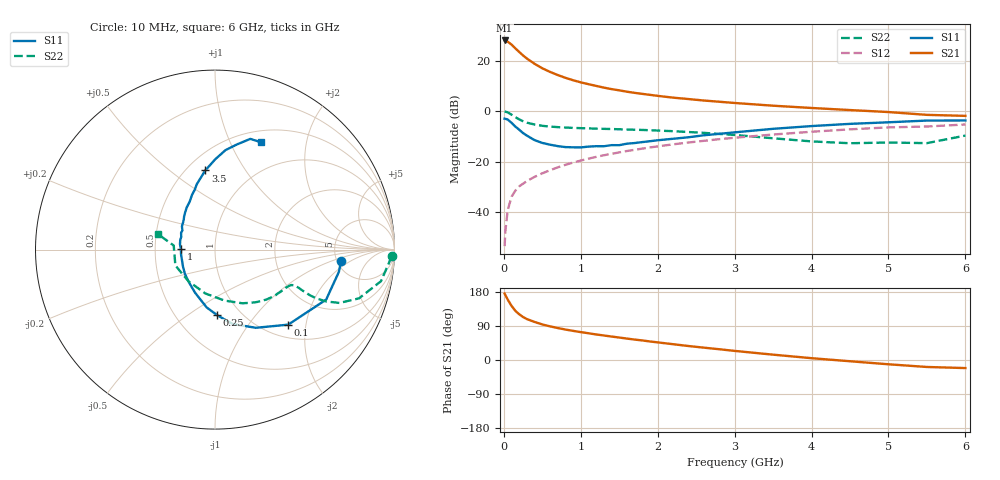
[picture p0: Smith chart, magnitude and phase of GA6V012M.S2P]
! Infineon Technologies  Discrete & RF Semiconductors
! BF775
! Si NPN RF Bipolar Junction Transistor in SOT23
! VCE = 6 V  IC = 12 mA
! Common Emitter S-Parameters:  May  1996
# GHz  S  MA  R  50
!  f  S11  S21  S12  S22
! GHz  MAG  ANG  MAG  ANG  MAG  ANG  MAG  ANG
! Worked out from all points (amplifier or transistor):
!   36 points, 10 MHz to 6 GHz, reference 50 ohm
!   highest |S21| = 28.0 dB at 10 MHz (marker M1)
!   |S21| within 3 dB of that: start of sweep to 145.3 MHz
!   unconditionally stable (mu >= 1): 552.3 MHz to 2.917 GHz
!   at 250 MHz: K = 0.72, MSG = 25.4 dB, |S12| = -28.8 dB
!   at 1.4 GHz: K = 1.10, MAG = 10.9 dB, |S12| = -17.0 dB
!   at 6 GHz: K = 0.91, MSG = 1.7 dB, |S12| = -5.3 dB
!   S11 on the Smith chart (normalised r, x): 10 MHz: 5.42, -1.38; 100 MHz: 1.25, -1.59; 250 MHz: 0.78, -0.66; 1 GHz: 0.68, +0.00; 3.5 GHz: 0.61, +0.68; 6 GHz: 0.63, +1.31
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0.01  0.7051 -5.2  25.04 175.4  0.0021 89.7  0.9842 -2.2
0.02  0.7013 -10.2  24.7 171.1  0.0042 86.2  0.9713 -4.5
0.05  0.6791 -24.2  23.7 159.6  0.0108 79.8  0.9413 -10.8
0.1  0.5842 -45.7  20.73 142.9  0.02 71.4  0.8471 -18.7
0.15  0.4916 -62.4  17.44 129.7  0.0265 66.1  0.7544 -23.2
0.2  0.426 -76.7  14.8 120.6  0.0322 64.3  0.6837 -25.0
0.25  0.3661 -88.0  12.64 113.4  0.0363 63.2  0.6273 -25.7
0.3  0.3255 -98.2  10.97 108.0  0.0411 63.8  0.5882 -25.7
0.4  0.2649 -114.7  8.622 100.4  0.0496 64.7  0.5401 -25.1
0.5  0.2332 -128.5  7.033 93.8  0.0583 66.0  0.5098 -24.5
0.6  0.2156 -141.0  5.97 88.8  0.0671 66.8  0.4918 -24.3
0.7  0.2019 -152.0  5.175 84.4  0.0765 67.1  0.4799 -24.5
0.8  0.193 -162.6  4.556 80.4  0.0859 66.9  0.4707 -24.8
1  0.1901 179.1  3.705 73.6  0.1045 66.6  0.4581 -26.3
1.1  0.1973 171.3  3.405 70.6  0.1139 66.4  0.4526 -27.5
1.3  0.2008 159.6  2.912 64.7  0.133 65.2  0.4436 -29.6
1.6  0.2257 144.7  2.415 56.5  0.1614 63.1  0.4304 -33.9
2.2  0.2822 124.1  1.842 41.7  0.2188 57.7  0.3987 -44.3
3.5  0.4444 97.0  1.276 14.1  0.3424 43.1  0.2886 -79.6
4.5  0.5571 84.0  1.046 -3.3  0.434 30.4  0.2301 -130.0
5.5  0.6476 72.3  0.84 -18.4  0.4937 15.5  0.2311 174.3
6  0.6503 67.0  0.802 -21.3  0.5415 11.4  0.3265 165.0
